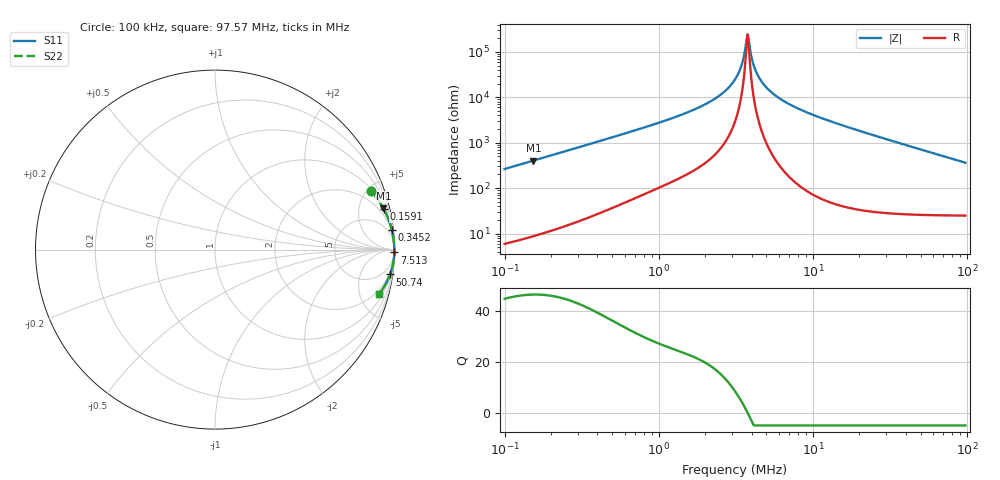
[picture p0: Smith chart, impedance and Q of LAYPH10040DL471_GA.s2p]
! LAYPH10040DL471_GA  S-PARAMETER MODEL  ( General Type )
! Model Generated by TAIYO YUDEN Corporation (http://www.ty-top.com)
! Version 1.0
! TAIYO YUDEN Control No. 180920NI43SB-FBB
! Copyright(c) 2018 TAIYO YUDEN CO.,LTD. All Rights Reserved.
! Product Description (link to TY-COMPAS)
! https://ds.yuden.co.jp/TYCOMPAS/or/detail?pn=LAYPH10040DL471MGA&u=M
! Products Name : Inductors
! Characteristics :
!  Inductance : 470 uH , SRF(min) : -Hz , DC Resistance(max) : 1.44 Ohm
!  Rated Current : Saturation :0.53 A , Temp Rise : 0.25 A (25 degC)
!  Case Size : 10.1 x 10.0 / 0.398 x 0.394 [mm/inch] , Thickness : 4 / 0.157 [mm/inch]
!  (Conditions: Temperature = 25 degC , DC Bias Current/Voltage = 0A / 0V)
! External Node Assignments :
!  1  o---GGG---o  2
! GND o---------o GND
! Frequency Range : 0.1MHz  -  97.572838MHz  [ 402 STEP ]
# MHz S RI R 50
! Freq[MHz].  S11 Real  S11 Imag  S21 Real  S21 Imag  S12 Real  S12 Imag  S22 Real  S22 Imag
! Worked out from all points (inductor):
!   401 points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, 100 kHz to 97.57 MHz, reference 50 ohm
!   read as one part in series: L = 418 uH near 103.5 kHz
!   highest Q = 46.3 at 153.8 kHz (marker M1), where L = 418 uH
!   self-resonance near 3.71 MHz
!   S11 on the Smith chart (normalised r, x): 100 kHz: 1.12, +5.27; 159.1 kHz: 1.18, +8.36; 345.2 kHz: 1, +18; 7.513 MHz: open; 50.74 MHz: 2, -14; 97.57 MHz: 1.50, -7.24
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0.1  0.8686 0.3268  0.1314 -0.3268  0.1314 -0.3268  0.8686 0.3268
0.153756  0.9378 0.2309  0.0622 -0.2309  0.0622 -0.2309  0.9378 0.2309
0.15914  0.9415 0.2241  0.0585 -0.2241  0.0585 -0.2241  0.9415 0.2241
0.316747  0.983 0.118  0.017 -0.118  0.017 -0.118  0.983 0.118
0.345207  0.9854 0.1085  0.0146 -0.1085  0.0146 -0.1085  0.9854 0.1085
1.003287  0.9974 0.0361  0.00264 -0.0361  0.00264 -0.0361  0.9974 0.0361
2.17633  0.9992 0.0122  0.000816 -0.0122  0.000816 -0.0122  0.9992 0.0122
2.721936  0.9994 0.00702  0.000587 -0.00702  0.000587 -0.00702  0.9994 0.00702
3.177882  0.9995 0.00364  0.000483 -0.00364  0.000483 -0.00364  0.9995 0.00364
3.404326  0.9996 0.00217  0.000449 -0.00217  0.000449 -0.00217  0.9996 0.00217
3.646904  0.9996 0.00071  0.000423 -0.00071  0.000423 -0.00071  0.9996 0.00071
3.774601  0.9996 -2.1e-05  0.000412 2.1e-05  0.000412 2.1e-05  0.9996 -2.1e-05
3.906768  0.9996 -0.000752  0.000404 0.000752  0.000404 0.000752  0.9996 -0.000752
4.043564  0.9996 -0.00149  0.000397 0.00149  0.000397 0.00149  0.9996 -0.00149
4.185149  0.9996 -0.00222  0.000392 0.00222  0.000392 0.00222  0.9996 -0.00222
4.720894  0.9996 -0.00482  0.000389 0.00482  0.000389 0.00482  0.9996 -0.00482
5.704673  0.9996 -0.00907  0.000431 0.00907  0.000431 0.00907  0.9996 -0.00907
7.512836  0.9994 -0.0159  0.000612 0.0159  0.000612 0.0159  0.9994 -0.0159
9.894118  0.999 -0.0239  0.000992 0.0239  0.000992 0.0239  0.999 -0.0239
31.33933  0.9903 -0.0864  0.00967 0.0864  0.00967 0.0864  0.9903 -0.0864
50.73909  0.9751 -0.1385  0.0249 0.1385  0.0249 0.1385  0.9751 -0.1385
97.57284  0.915 -0.2468  0.085 0.2468  0.085 0.2468  0.915 -0.2468
